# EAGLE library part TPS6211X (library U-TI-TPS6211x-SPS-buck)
TPS6211x 17-V, 1.5-A, Synchronous Step-Down Converter
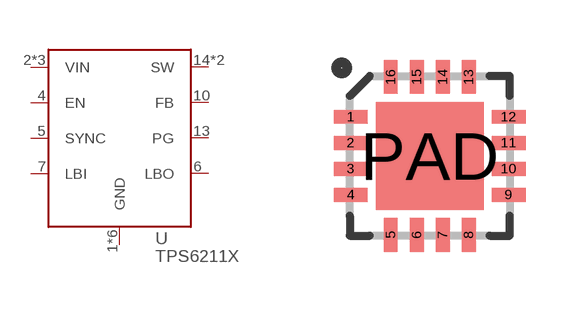
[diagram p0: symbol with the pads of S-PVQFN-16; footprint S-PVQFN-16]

Designator prefix U

## TPS6211X  [S-PVQFN-16]
1  GND  pwr
2  VIN  pwr
3  VIN  pwr
4  EN  in
5  SYNC  in
6  LBO  oc
7  LBI  in
8  VIN  pwr
9  GND  pwr
10  FB  in
11  GND  pwr
12  GND  pwr
13  PG  oc
14  SW  out
15  SW  out
16  GND  pwr
PAD  GND  pwr

## Footprint S-PVQFN-16 (pad centres in mm)
smd 0.85 x 0.35: 1 -1.975,0.975; 2 -1.975,0.325; 3 -1.975,-0.325; 4 -1.975,-0.975; 9 1.975,-0.975; 10 1.975,-0.325; 11 1.975,0.325; 12 1.975,0.975
smd 0.35 x 0.85: 5 -0.975,-1.975; 6 -0.325,-1.975; 7 0.325,-1.975; 8 0.975,-1.975; 13 0.975,1.975; 14 0.325,1.975; 15 -0.325,1.975; 16 -0.975,1.975
smd 2.7 x 2.7: PAD 0,0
